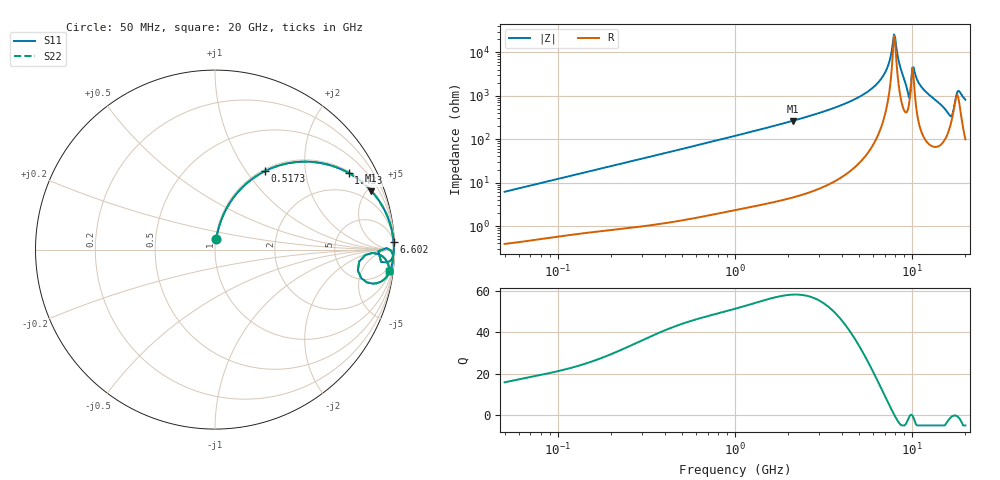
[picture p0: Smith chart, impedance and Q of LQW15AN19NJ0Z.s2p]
!Murata Part Number: LQW15AN19NJ0Z
!These Parameters are Measured in Series Mode Connection
!  o--[Z]--o
!Port1  Port2
!  o-------o
!Freq. Start=50[MHz] Stop=20[GHz], 401[Steps]
# Hz S RI R 50
!Freq.(Hz) S11(Real) S11(Imag) S21(Real) S21(Imag) S12(Real) S12(Imag) S22(Real) S22(Imag)
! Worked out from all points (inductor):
!   401 points, 50 MHz to 20 GHz, reference 50 ohm
!   read as one part in series: L = 19.5 nH near 51.52 MHz
!   highest Q = 58.2 at 2.115 GHz (marker M1), where L = 19.9 nH
!   self-resonance near 7.902 GHz
!   S11 on the Smith chart (normalised r, x): 50 MHz: 1.01, +0.12; 517.3 MHz: 1.03, +1.23; 1.433 GHz: 1.06, +3.45; 6.602 GHz: 4, +46; 20 GHz: 3, -16
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5e7  0.0076 0.0608  0.9924 -0.0608  0.9924 -0.0608  0.0076 0.0608
1.364002e8  0.0325 0.1578  0.9675 -0.1578  0.9675 -0.1578  0.0325 0.1578
3.721004e8  0.1697 0.363  0.8303 -0.363  0.8303 -0.363  0.1697 0.363
5.173368e8  0.2782 0.437  0.7218 -0.437  0.7218 -0.437  0.2782 0.437
1e9  0.585 0.4831  0.415 -0.4831  0.415 -0.4831  0.585 0.4831
1.432596e9  0.7452 0.4268  0.2548 -0.4268  0.2548 -0.4268  0.7452 0.4268
2.114743e9  0.8703 0.3275  0.1297 -0.3275  0.1297 -0.3275  0.8703 0.3275
2.728004e9  0.9233 0.2574  0.0767 -0.2574  0.0767 -0.2574  0.9233 0.2574
4.81993e9  0.9835 0.1143  0.0165 -0.1143  0.0165 -0.1143  0.9835 0.1143
6.601595e9  0.995 0.0433  0.005 -0.0433  0.005 -0.0433  0.995 0.0433
7.442007e9  0.9964 0.0159  0.00359 -0.0159  0.00359 -0.0159  0.9964 0.0159
7.784049e9  0.9964 0.00508  0.00356 -0.00508  0.00356 -0.00508  0.9964 0.00508
8.020766e9  0.9962 -0.00246  0.00376 0.00246  0.00376 0.00246  0.9962 -0.00246
8.644534e9  0.9944 -0.0239  0.00565 0.0239  0.00565 0.0239  0.9944 -0.0239
9.457416e9  0.9636 -0.071  0.0364 0.071  0.0364 0.071  0.9636 -0.071
1.019291e10  0.9863 -0.0171  0.0137 0.0171  0.0137 0.0171  0.9863 -0.0171
1.034674e10  0.9895 -0.0266  0.0105 0.0266  0.0105 0.0266  0.9895 -0.0266
1.166392e10  0.989 -0.0718  0.011 0.0718  0.011 0.0718  0.989 -0.0718
1.621653e10  0.8469 -0.1826  0.1531 0.1826  0.1531 0.1826  0.8469 -0.1826
1.670968e10  0.7957 -0.1173  0.2043 0.1173  0.2043 0.1173  0.7957 -0.1173
1.828096e10  0.9482 -0.0516  0.0518 0.0516  0.0518 0.0516  0.9482 -0.0516
2e10  0.9707 -0.1176  0.0293 0.1176  0.0293 0.1176  0.9707 -0.1176
